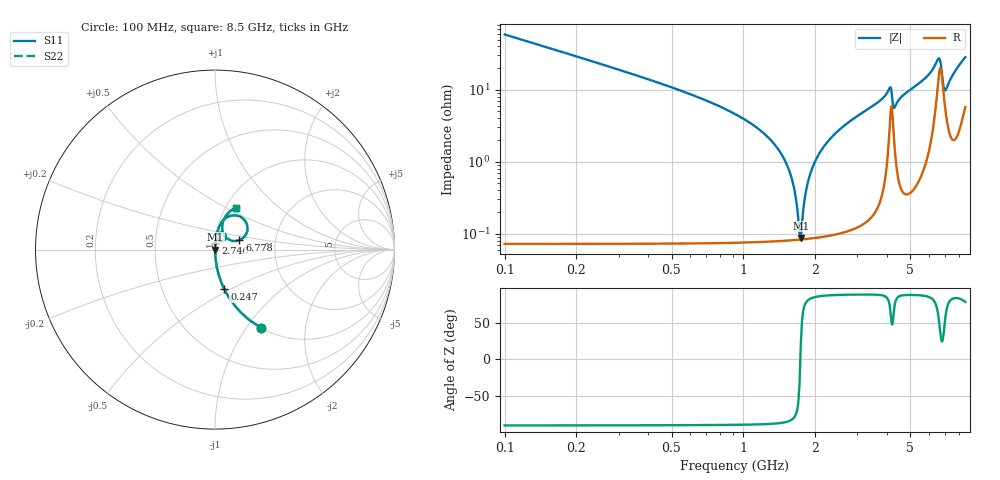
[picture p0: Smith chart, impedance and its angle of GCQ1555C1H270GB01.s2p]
!Murata Part Number: GCQ1555C1H270GB01
!These Parameters are Measured in Series Mode Connection
!Data Generated on Jan 08, 2026
!  o--ll--o
!Port1  Port2
!  o------o
!Operation Temp=25[degC], DC Bias Voltage=0[V]
!Freq. Start=100[MHz] Stop=9[GHz] 401[Steps]
# Hz S RI R 50
!Freq.(Hz) S11(Real) S11(Imag) S21(Real) S21(Imag) S12(Real) S12(Imag) S22(Real) S22(Imag)
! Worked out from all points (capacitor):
!   401 points, 100 MHz to 8.5 GHz, reference 50 ohm
!   read as one part in series: C = 27 pF near 142 MHz
!   lowest |Z| = 87.3 mohm at 1.738 GHz (marker M1)
!   series resonance near 1.731 GHz, so ESL is about 310 pH
!   S11 on the Smith chart (normalised r, x): 100 MHz: 1.00, -1.18; 247 MHz: 1.00, -0.47; 2.746 GHz: 1.00, +0.07; 6.778 GHz: 1.31, +0.14; 8.5 GHz: 1.12, +0.56
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1e8  0.2569 -0.4363  0.7431 0.4363  0.7431 0.4363  0.2569 -0.4363
2.47e8  0.0525 -0.2215  0.9475 0.2215  0.9475 0.2215  0.0525 -0.2215
5.2e8  0.0113 -0.1021  0.9887 0.1021  0.9887 0.1021  0.0113 -0.1021
1.255e9  0.00128 -0.0225  0.9987 0.0225  0.9987 0.0225  0.00128 -0.0225
1.507e9  0.000891 -0.00964  0.9991 0.00964  0.9991 0.00964  0.000891 -0.00964
1.612e9  0.000835 -0.00496  0.9992 0.00496  0.9992 0.00496  0.000835 -0.00496
1.696e9  0.000824 -0.00143  0.9992 0.00143  0.9992 0.00143  0.000824 -0.00143
1.738e9  0.000828 0.000274  0.9992 -0.000274  0.9992 -0.000274  0.000828 0.000274
1.864e9  0.000874 0.00518  0.9991 -0.00518  0.9991 -0.00518  0.000874 0.00518
2.032e9  0.00101 0.0113  0.999 -0.0113  0.999 -0.0113  0.00101 0.0113
2.305e9  0.00137 0.0207  0.9986 -0.0207  0.9986 -0.0207  0.00137 0.0207
2.746e9  0.0023 0.0349  0.9977 -0.0349  0.9977 -0.0349  0.0023 0.0349
2.914e9  0.00279 0.0402  0.9972 -0.0402  0.9972 -0.0402  0.00279 0.0402
4.09e9  0.0366 0.0953  0.9634 -0.0953  0.9634 -0.0953  0.0366 0.0953
4.3e9  0.0181 0.0535  0.9819 -0.0535  0.9819 -0.0535  0.0181 0.0535
4.657e9  0.0106 0.0823  0.9894 -0.0823  0.9894 -0.0823  0.0106 0.0823
5.707e9  0.0268 0.1355  0.9732 -0.1355  0.9732 -0.1355  0.0268 0.1355
6.547e9  0.1553 0.1738  0.8447 -0.1738  0.8447 -0.1738  0.1553 0.1738
6.778e9  0.1357 0.0521  0.8643 -0.0521  0.8643 -0.0521  0.1357 0.0521
6.925e9  0.0733 0.0585  0.9267 -0.0585  0.9267 -0.0585  0.0733 0.0585
7.114e9  0.0447 0.0938  0.9553 -0.0938  0.9553 -0.0938  0.0447 0.0938
8.5e9  0.1156 0.2323  0.8844 -0.2323  0.8844 -0.2323  0.1156 0.2323
